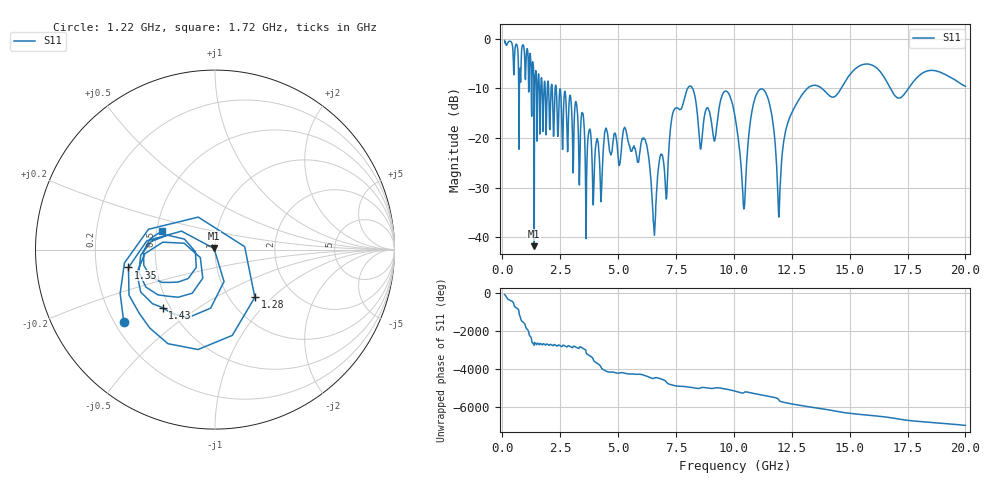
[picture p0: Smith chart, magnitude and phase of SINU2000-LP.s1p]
!Keysight Technologies,P9374A,MY57211922,A.15.40.13
!Date: Friday, July 10, 2026 13:41:02
!Correction: S11(C  1-Port  )
!S1P File: Measurement: S11:
# Hz S  dB  R 50
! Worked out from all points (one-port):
!   1991 points, 100 MHz to 20 GHz, reference 50 ohm
!   lowest |S11| = -41.8 dB at 1.38 GHz (marker M1), VSWR 1.02, Z = 49.5 + j0.617 ohm
!   |S11| at or under -10 dB: 2.329 GHz to 8.008 GHz (5.678 GHz wide, 110 % of centre); 8.22 GHz to 13.17 GHz (4.951 GHz wide, 46.3 % of centre); 13.81 GHz to 14.64 GHz (829.8 MHz wide, 5.84 % of centre)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
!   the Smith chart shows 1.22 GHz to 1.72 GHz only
!   S11 on the Smith chart (normalised r, x): 1.22 GHz: 0.24, -0.33; 1.28 GHz: 1.30, -0.79; 1.35 GHz: 0.34, -0.09; 1.43 GHz: 0.46, -0.37; 1.72 GHz: 0.54, +0.12
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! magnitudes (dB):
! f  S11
! 100 MHz  -0.3
! 1.22 GHz  -3.8
! 1.28 GHz  -9.2
! 1.35 GHz  -6.2
! 1.38 GHz  -41.8
! 1.43 GHz  -7.2
! 1.72 GHz  -10.1
! 2.59 GHz  -20.9
! 3.47 GHz  -15.0
! 3.94 GHz  -31.9
! 4.48 GHz  -18.0
! 5.08 GHz  -25.2
! 6.15 GHz  -20.2
! 6.56 GHz  -38.9
! 6.81 GHz  -23.9
! 7.09 GHz  -32.2
! 7.57 GHz  -13.9
! 8.18 GHz  -9.7
! 8.57 GHz  -22.2
! 10.05 GHz  -15.6
! 10.44 GHz  -34.2
! 10.83 GHz  -13.4
! 11.36 GHz  -10.7
! 11.95 GHz  -35.9
! 12.54 GHz  -14.6
! 15.03 GHz  -7.1
! 17.52 GHz  -10.1
! 20 GHz  -9.6
